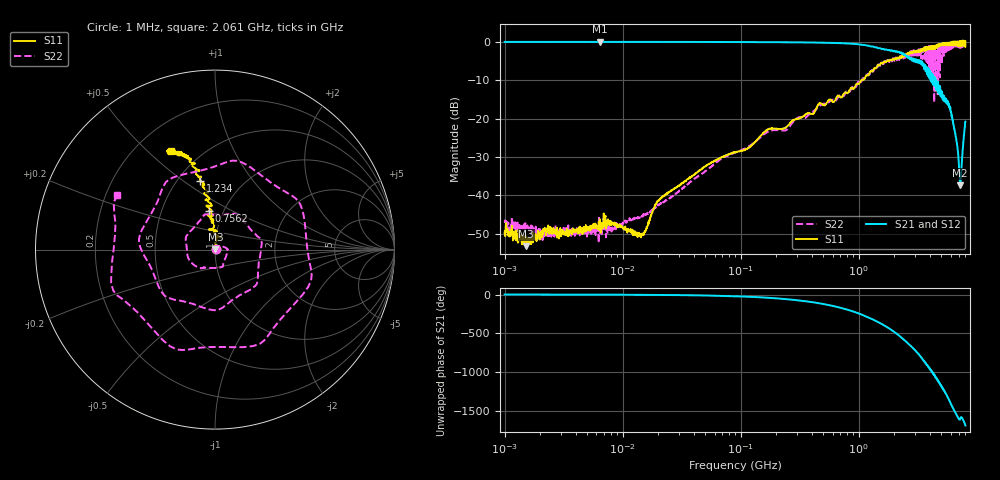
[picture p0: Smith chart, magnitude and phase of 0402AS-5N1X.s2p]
!s-Parameter Generated by FASTRON Sdn. Bhd.
!FASTRON P/N : 0402AS-5N1X
!Keysight Technologies: E5071C_MY46733604_B.14.02
!Date: Mon Dec 01 10:24:34 2025
!Version  :Rev00  Mon Dec 01 10:24:34 2025
!Data & Calibration Information:
!Freq  S11:SOLT2(ON)  S21:SOLT2(ON)  S12:SOLT2(ON)  S22:SOLT2(ON)
!PortZ  Port1:50+j0  Port2:50+j0
!When reading reference impedance value at option line is always used.
! Remarks : This data is being provided solely for informational purposes.
# Hz S dB R 50
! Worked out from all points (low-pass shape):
!   1601 points, 1 MHz to 8 GHz, reference 50 ohm
!   highest |S21| = 0.00 dB at 6.4 MHz (marker M1); lowest = -37.4 dB at 7.229 GHz (marker M2)
!   |S21| within 3 dB of the highest: start of sweep to 2.311 GHz
!   lowest |S11| = -53.2 dB at 1.523 MHz (marker M3), VSWR 1.00, Z = 50.2 + j0.119 ohm
!   |S11| at or under -10 dB: start of sweep to 1.052 GHz
!   |S22| runs from -52.4 to -0.4 dB; largest |S21 - S12| = 0.019
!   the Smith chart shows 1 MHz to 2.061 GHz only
!   S11 on the Smith chart (normalised r, x): 1 MHz: 1.01, +0.00; 756.2 MHz: 0.86, +0.38; 1.234 GHz: 0.64, +0.58; 2.061 GHz: 0.34, +0.59
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1000000  -49.70 31.6  -0.04 -0.2  -0.02 -0.2  -46.90 21.0
1522827  -53.20 32.9  -0.03 -0.4  -0.03 -0.4  -47.70 -6.4
4479405  -49.20 27.5  -0.05 -1.1  -0.03 -1.2  -49.90 35.0
6400096  -46.20 34.1  -0.00 -1.5  0.07 -2.0  -46.40 17.3
2.00676e7  -41.50 40.2  -0.05 -5.0  -0.04 -5.0  -42.50 63.8
8.994653e7  -28.70 89.8  -0.07 -22.3  -0.07 -22.2  -28.80 26.9
4.006501e8  -18.80 103.0  -0.20 -98.0  -0.19 -98.0  -18.40 -123.0
7.5621e8  -13.30 98.7  -0.41 175.0  -0.40 175.0  -13.90 74.1
1.233539e9  -8.11 102.0  -1.09 57.8  -1.09 57.8  -8.53 -167.0
1.473292e9  -6.11 104.0  -1.70 1.1  -1.69 1.0  -5.86 76.2
1.7949e9  -5.08 109.0  -2.11 -74.4  -2.11 -74.4  -5.15 -79.7
2.061212e9  -4.38 114.0  -2.61 -137.0  -2.60 -137.0  -4.12 151.0
2.340174e9  -3.65 120.0  -3.24 155.0  -3.22 154.0  -3.50 8.8
2.57493e9  -3.44 123.0  -3.66 98.1  -3.63 98.1  -3.74 -106.0
2.912392e9  -2.45 129.0  -5.10 19.3  -5.06 19.1  -2.58 83.2
3.26428e9  -2.67 137.0  -4.79 -64.6  -4.75 -64.9  -3.99 -85.3
3.60885e9  -1.89 146.0  -6.87 -144.0  -6.84 -144.0  -1.40 101.0
3.993958e9  -1.40 150.0  -9.47 127.0  -9.47 126.0  -2.11 -97.0
4.352635e9  -1.17 155.0  -11.30 37.1  -11.30 36.5  -15.80 109.0
5.528293e9  -0.42 -170.0  -16.00 148.0  -16.00 148.0  -1.87 -74.7
7.228903e9  0.12 -105.0  -37.40 -164.0  -37.50 -164.0  -1.20 170.0
8e9  0.11 -92.3  -20.80 110.0  -20.80 109.0  -1.29 156.0
